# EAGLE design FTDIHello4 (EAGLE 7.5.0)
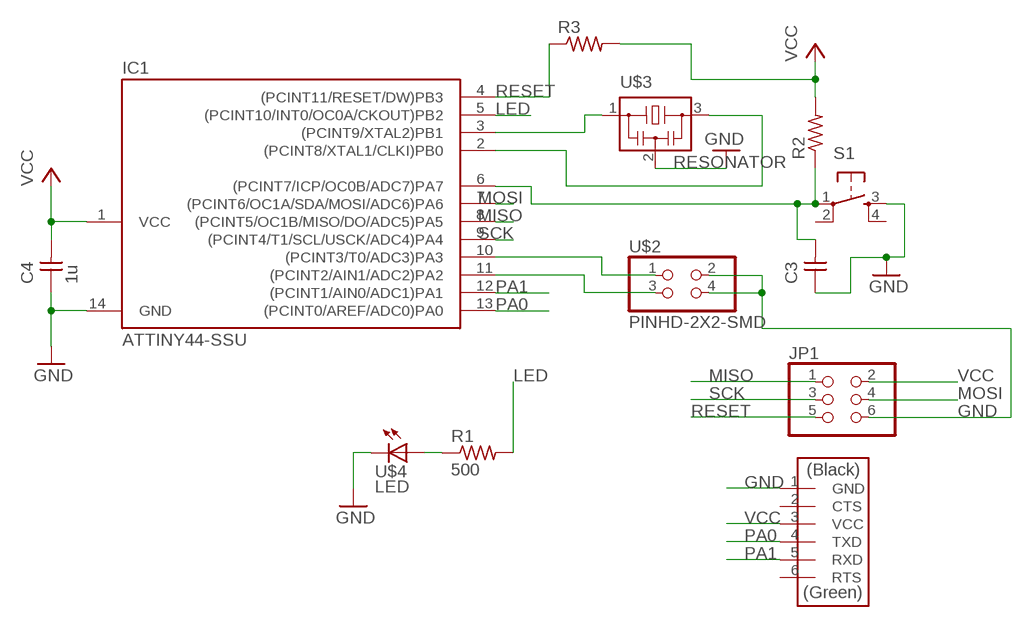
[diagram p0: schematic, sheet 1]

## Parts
C3  CAP-UNPOLARIZEDFAB  [C1206FAB]
C4  1u  CAP-UNPOLARIZEDFAB  [C1206FAB]
IC1  ATTINY44-SSU  [SOIC14]
JP1  PINHD-2X3-SMD  [2X03SMD]
R1  500  RES-US1206FAB  [R1206FAB]
R2  RES-US1206FAB  [R1206FAB]
R3  RES-US1206FAB  [R1206FAB]
S1  6MM_SWITCH6MM_SWITCH  [6MM_SWITCH]
U$1  FTDI-SMD-HEADER  [1X06SMD]
U$2  PINHD-2X2-SMD  [2X02SMD]
U$3  RESONATOR  [EFOBM]
U$4  LED  [LED1206]

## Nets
GND: C3.1 C4.1 IC1.14(GND) JP1.6 S1.3(S) U$1.1(GND) U$2.2 U$2.4 U$3.2 U$4.2(C)
LED: IC1.5((PCINT10/INT0/OC0A/CKOUT)PB2) R1.2
MISO: IC1.8((PCINT5/OC1B/MISO/DO/ADC5)PA5) JP1.1
MOSI: IC1.7((PCINT6/OC1A/SDA/MOSI/ADC6)PA6) JP1.4
N$1: IC1.3((PCINT9/XTAL2)PB1) U$3.1
N$2: IC1.2((PCINT8/XTAL1/CLKI)PB0) U$3.3
N$3: R1.1 U$4.1(A)
N$4: C3.2 IC1.6((PCINT7/ICP/OC0B/ADC7)PA7) R2.1 S1.1(P)
N$6: IC1.10((PCINT3/T0/ADC3)PA3) U$2.1
N$7: IC1.11((PCINT2/AIN1/ADC2)PA2) U$2.3
PA0: IC1.13((PCINT0/AREF/ADC0)PA0) U$1.4(TXD)
PA1: IC1.12((PCINT1/AIN0/ADC1)PA1) U$1.5(RXD)
RESET: IC1.4((PCINT11/RESET/DW)PB3) JP1.5 R3.1
SCK: IC1.9((PCINT4/T1/SCL/USCK/ADC4)PA4) JP1.3
VCC: C4.2 IC1.1(VCC) JP1.2 R2.2 R3.2 U$1.3(VCC)
Unconnected: S1.2(P1) S1.4(S1) U$1.2(CTS) U$1.6(RTS)

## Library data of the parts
C3 C4 = fab:CAP-UNPOLARIZED
IC1 = fab:ATTINY44
JP1 = fab:PINHD-2X3-SMD: PIN HEADER
R1-R3 = fab:RES-US: Resistor (US Symbol)
S1 = fab:6MM_SWITCH: OMRON SWITCH
U$1 = fab:FTDI-SMD-HEADER
U$2 = fab:PINHD-2X2-SMD
U$3 = fab:RESONATOR
U$4 = fab:LED: LED

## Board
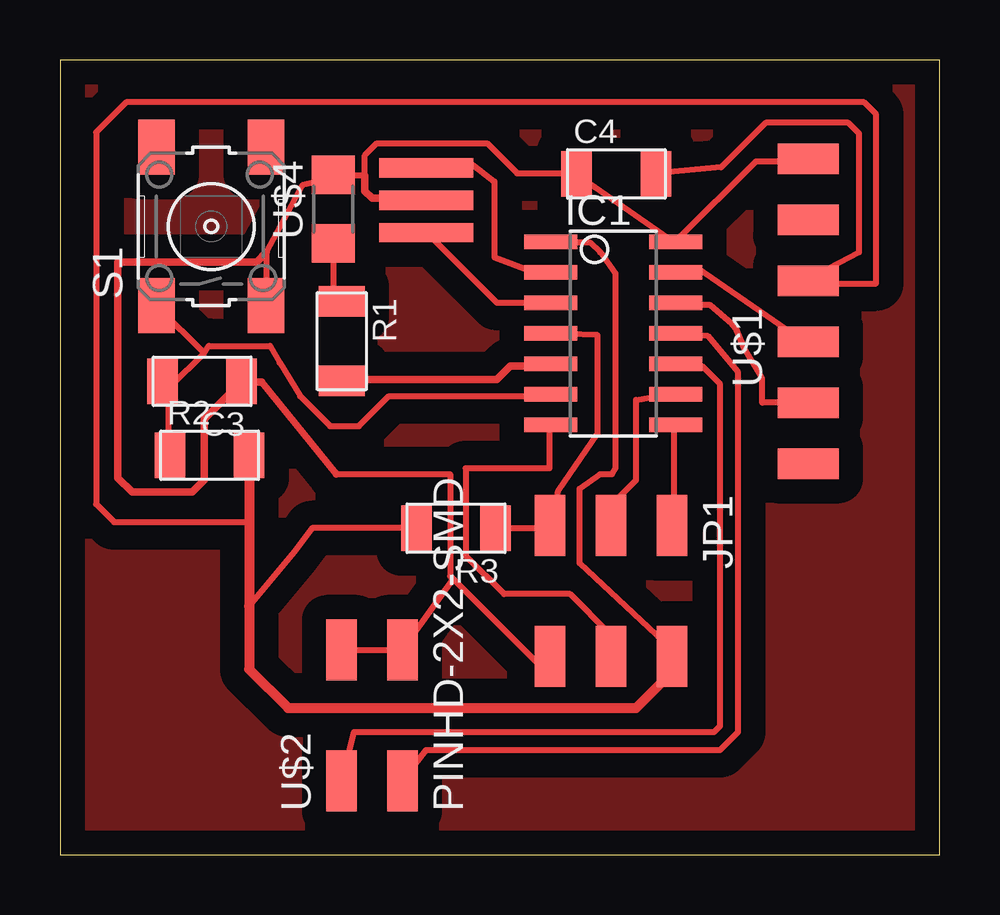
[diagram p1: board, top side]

Size 36.65 x 33.14 mm. Coordinates in mm from the lower left corner, seen from the top.
Outline: 0,0 36.65,0 36.65,33.14 0,33.14 0,0
Copper layers (1*16): Top 0.035mm / dielectric 1.5mm / Bottom 0.035mm
Design rules "default *": minimum track width 10mil, minimum drill 24mil, track to track 15mil, track to pad 15mil, pad to pad 15mil, via to via 8mil, smd to smd 15mil, copper to edge 40mil, drill to drill 8mil, minimum pad ring 10mil, minimum via ring 8mil, stop-mask expansion 4mil, vias tented up to drill 0mil, thermal gap 10mil

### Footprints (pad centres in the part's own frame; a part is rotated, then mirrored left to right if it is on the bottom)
C1206FAB = smd 1.27 x 1.905: 1 -1.651,0; 2 1.651,0
SOIC14 = smd 0.61 x 2.21: 1 -3.81,-2.603; 2 -2.54,-2.603; 3 -1.27,-2.603; 4 0,-2.603; 5 1.27,-2.603; 6 2.54,-2.603; 7 3.81,-2.603; 8 3.81,2.603; 9 2.54,2.603; 10 1.27,2.603; 11 0,2.603; 12 -1.27,2.603; 13 -2.54,2.603; 14 -3.81,2.603
2X03SMD = smd 2.54 x 1.27: 1 -2.54,2.54; 2 2.92,2.54; 3 -2.54,0; 4 2.92,0; 5 -2.54,-2.54; 6 2.92,-2.54
R1206FAB = smd 1.27 x 1.905: 1 -1.651,0; 2 1.651,0
6MM_SWITCH = smd 2.286 x 1.524: 1 -3.302,2.286; 2 3.302,2.286; 3 -3.302,-2.286; 4 3.302,-2.286
1X06SMD = smd 2.54 x 1.27: 1 0,6.35; 2 0,3.81; 3 0,1.27; 4 0,-1.27; 5 0,-3.81; 6 0,-6.35
2X02SMD = smd 2.54 x 1.27: 1 -2.54,1.27; 2 2.92,1.27; 3 -2.54,-1.27; 4 2.92,-1.27
EFOBM = smd 0.8 x 3.9: 1 -1.35,0; 2 0,0; 3 1.35,0
LED1206 = smd 1.6 x 1.803: 1 -1.422,0; 2 1.422,0

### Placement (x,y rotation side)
C3  5.92,19.74 180 top
C4  23.18,28.39 0 top
IC1  23.05,21.74 270 top
JP1  22.96,11.19 270 top
R1  11.74,21.42 270 top
R2  6.23,16.66 0 top
R3  16.5,13.62 180 top
S1  6.3,26.2 90 top
U$1  31.17,22.66 0 top
U$2  13,5.62 90 top
U$3  15.26,27.29 90 top
U$4  11.39,26.92 90 top

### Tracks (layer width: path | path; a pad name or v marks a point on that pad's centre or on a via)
GND
  Top 0.254: 7.6,19.72 C3.1 7.6,19.62 | 20.4,8.32 JP1.6 20.25,8.1 20.25,7.62 16.38,11.49 | U$1.1 31.1,28.92 29,28.92 25.7,25.62 IC1.14 25.6,25.52 22.3,27.82 21.6,28.32 C4.1 21.5,28.42 19.05,28.42 17.8,29.67 13.2,29.67 12.7,29.17 12.7,28.32 11.4,28.32 U$4.2 11.4,28.22 10.1,27.92 8.6,25.12 8.6,22.92 S1.3 | 13.7,27.32 15.2,27.32 U$3.2 | 11.5,15.87 16.25,15.87 16.25,11.62 16.38,11.49 | 16.38,11.49 U$2.4 U$2.2
  Top 0.305: C3.1 6,18.17 6,15.62 5.5,15.12 3,15.12 2.4,15.72 2.4,24.72 8.2,24.72 8.6,25.12 | 7.6,19.72 8.4,19.72 11.5,15.87 | 12.7,28.32 12.7,27.67 13,27.37 13.65,27.37 13.7,27.32
LED
  Top 0.254: 19.7,20.42 20.4,20.42 IC1.5 | 11.8,19.82 R1.2
  Top 0.305: 11.8,19.82 18.2,19.82 18.75,20.37 19.65,20.37 19.7,20.42
MISO
  Top 0.254: IC1.8 25.6,17.92 25.6,13.92 25.5,13.82 JP1.1
MOSI
  Top 0.254: IC1.7 20.4,17.92 20.4,16.12 16.9,16.12 16.9,12.47 18.5,10.87 21.25,10.87 22.9,9.22 22.9,8.82 JP1.4
N$1
  Top 0.254: IC1.3 20.4,23.02 18.2,23.02 15.3,25.92 U$3.1
N$2
  Top 0.254: IC1.2 20.4,24.32 19.7,24.32 18.1,24.92 18.1,28.07 17.05,28.87 15.3,28.62 U$3.3
N$3
  Top 0.254: U$4.1 11.4,25.42 11.4,23.42 11.7,23.12 R1.1
N$4
  Top 0.254: R2.1 4.5,16.72 4.5,19.52 4.3,19.72 C3.2 4.6,19.52 6,20.92 | 6,20.92 6.2,21.22 8.75,21.22 9.15,20.52 10,19.12 11.25,17.87 12.45,17.87 13.7,19.12 20.4,19.12 IC1.6 | 6,20.92 4.1,22.82 S1.1
N$5
  pour Top (isolate 1.016): 0,33.37 36.75,33.37 36.75,-0.38 0,-0.13
N$6
  Top 0.254: U$2.1 12.25,5.12 27.25,5.12 27.5,5.37 27.5,19.62 26.75,20.37 IC1.10
N$7
  Top 0.254: U$2.3 15.25,4.37 27.5,4.37 28.25,5.12 28.25,20.12 27,21.62 IC1.11
PA0
  Top 0.254: IC1.13 25.7,24.22 26.55,24.47 30.6,21.67 U$1.4
PA1
  Top 0.254: IC1.12 25.7,22.92 27.1,22.92 28,22.12 28.2,21.87 28.5,21.12 29.25,19.87 29.25,18.87 29.27,18.85 U$1.5
RESET
  Top 0.254: IC1.4 20.5,21.72 21.1,21.72 22.4,21.67 22.4,17.57 20.75,15.17 20.5,13.82 JP1.5 20.31,13.62 R3.1
SCK
  Top 0.254: IC1.9 25.6,19.12 24.9,19.12 24,18.97 24,15.62 23,14.62 23,13.82 JP1.3
VCC
  Top 0.254: C4.2 24.9,28.42 27.55,28.67 29.4,30.52 32.85,30.52 33.3,30.07 33.3,25.12 31.2,24.02 U$1.3 31.2,23.82 34,23.82 34,30.87 33.5,31.37 2.75,31.37 1.5,30.12 1.5,14.62 2.25,13.87 7.88,13.87 | IC1.1 20.5,25.52 22.1,25.52 22.5,25.12 23.15,24.22 23.15,16.12 23,15.87 22.5,15.87 21.65,15.27 21.65,12.17 25.5,8.57 JP1.2 | R3.2 10.5,13.62 9.75,12.62 7.88,10.37
  Top 0.406: R2.2 7.88,13.87 7.88,10.37 7.88,7.74 9.5,6.12 24,6.12 25.5,7.62 JP1.2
